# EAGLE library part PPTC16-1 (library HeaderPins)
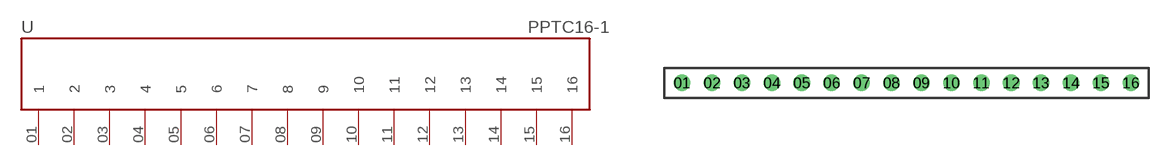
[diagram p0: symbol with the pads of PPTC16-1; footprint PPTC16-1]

Designator prefix -

## PPTC16-1LFBN-RC  [PPTC16-1]
01  1
02  2
03  3
04  4
05  5
06  6
07  7
08  8
09  9
10  10
11  11
12  12
13  13
14  14
15  15
16  16

## Footprint PPTC16-1 (pad centres in mm)
drill 0.9 pad 1.27: 01 -19.05,0; 02 -16.51,0; 03 -13.97,0; 04 -11.43,0; 05 -8.89,0; 06 -6.35,0; 07 -3.81,0; 08 -1.27,0; 09 1.27,0; 10 3.81,0; 11 6.35,0; 12 8.89,0; 13 11.43,0; 14 13.97,0; 15 16.51,0; 16 19.05,0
